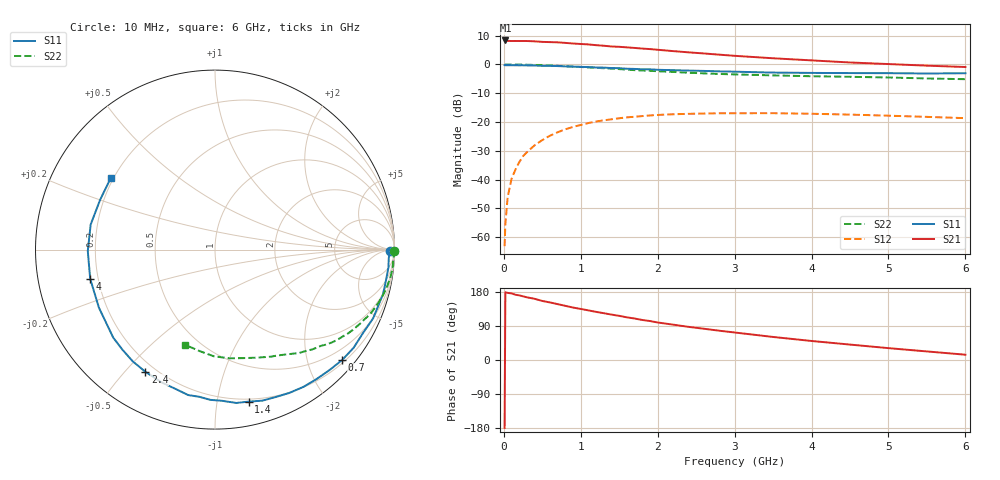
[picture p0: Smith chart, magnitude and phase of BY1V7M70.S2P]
! SIEMENS Small Signal Semiconductors
! BFY420
! Si NPN RF SIEGET Grounded Emitter Transistor in MICRO-X
! VCE = 1.75 V  IC = 0.7 mA
! Common Emitter S-Parameters:  October  1996
# GHz  S  MA  R  50
!  f  S11  S21  S12  S22
! GHz  MAG  ANG  MAG  ANG  MAG  ANG  MAG  ANG
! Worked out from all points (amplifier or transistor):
!   36 points, 10 MHz to 6 GHz, reference 50 ohm
!   highest |S21| = 8.3 dB at 20 MHz (marker M1)
!   |S21| within 3 dB of that: start of sweep to 1.902 GHz
!   unconditionally stable (mu >= 1): 4.719 GHz to end of sweep
!   at 250 MHz: K = 0.04, MSG = 20.0 dB, |S12| = -31.8 dB
!   at 1.4 GHz: K = 0.19, MSG = 12.6 dB, |S12| = -19.0 dB
!   at 6 GHz: K = 1.38, MAG = 5.2 dB, |S12| = -18.6 dB
!   S11 on the Smith chart (normalised r, x): 10 MHz: 69, -23; 700 MHz: 0.26, -2.65; 1.4 GHz: 0.18, -1.23; 2.4 GHz: 0.16, -0.57; 4 GHz: 0.17, -0.11; 6 GHz: 0.19, +0.30
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0.01  0.9745 -0.5  2.601 -179.2  0.0007 103.9  0.9999 -0.4
0.02  0.9716 -1.4  2.613 178.8  0.0017 92.1  0.9955 -0.6
0.05  0.9693 -2.9  2.571 177.1  0.005 90.4  0.998 -1.5
0.1  0.9715 -5.9  2.556 175.8  0.0103 87.8  0.9941 -3.0
0.15  0.9686 -8.7  2.559 172.2  0.0149 84.2  0.9939 -4.5
0.2  0.9678 -11.8  2.555 170.6  0.0201 83.2  0.9951 -5.8
0.3  0.9632 -17.7  2.555 165.4  0.03 79.2  0.9897 -8.8
0.4  0.9607 -23.5  2.524 161.5  0.0395 74.9  0.9816 -11.8
0.5  0.9466 -29.4  2.468 155.8  0.0487 71.7  0.9719 -14.6
0.7  0.9382 -41.0  2.423 147.4  0.0666 64.7  0.9482 -20.0
0.9  0.9166 -52.0  2.313 138.4  0.0824 57.3  0.9187 -25.1
1.1  0.8993 -62.7  2.23 130.9  0.0963 50.8  0.8902 -30.0
1.4  0.8675 -77.5  2.053 119.8  0.1118 42.1  0.8468 -36.4
1.8  0.8249 -96.0  1.889 105.6  0.127 31.7  0.7873 -43.9
2.2  0.7968 -112.3  1.707 93.3  0.1367 22.7  0.7431 -50.8
2.4  0.7833 -119.7  1.625 87.5  0.139 19.1  0.7191 -53.9
2.8  0.7594 -132.8  1.481 77.3  0.1422 12.1  0.6843 -59.6
3.5  0.7232 -153.4  1.282 60.8  0.1426 2.9  0.6461 -68.7
4  0.7141 -166.9  1.178 50.2  0.1394 -2.3  0.6248 -75.4
4.5  0.7088 -179.4  1.083 40.7  0.1348 -6.7  0.611 -82.4
5.5  0.6976 156.5  0.954 22.6  0.1231 -11.4  0.5717 -98.7
6  0.7047 145.5  0.904 14.0  0.117 -11.5  0.5554 -107.8
